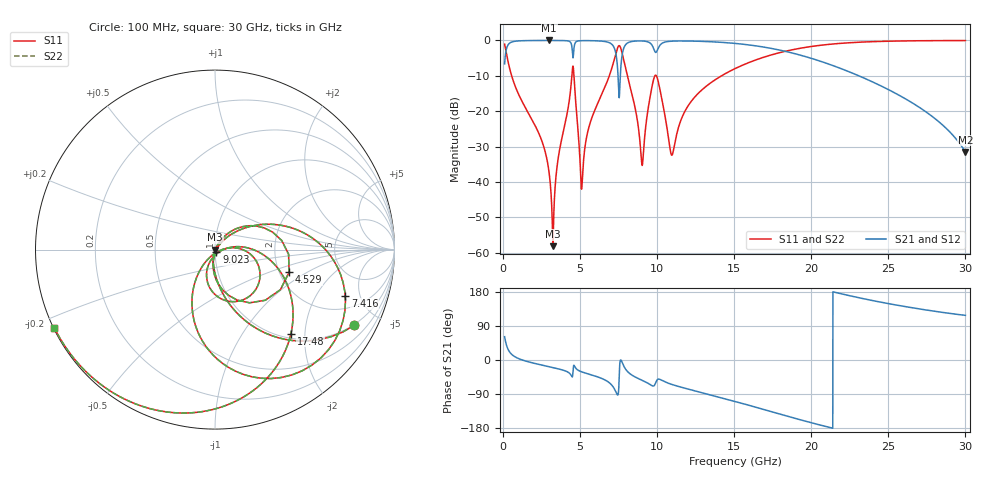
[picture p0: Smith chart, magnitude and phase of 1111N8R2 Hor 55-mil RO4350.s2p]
# GHz S MA R 50
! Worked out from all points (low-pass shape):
!   3201 points, 100 MHz to 30 GHz, reference 50 ohm
!   highest |S21| = -0.01 dB at 2.997 GHz (marker M1); lowest = -31.5 dB at 30 GHz (marker M2)
!   |S21| within 3 dB of the highest: 189.1 MHz to 4.496 GHz (4.307 GHz wide, 184 % of centre); 9.986 GHz to 18.24 GHz (8.255 GHz wide, 58.5 % of centre)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
!   lowest |S11| = -58.1 dB at 3.24 GHz (marker M3), VSWR 1.00, Z = 50.1 - j0.0199 ohm
!   |S11| at or under -10 dB: 557.3 MHz to 4.463 GHz (3.906 GHz wide, 156 % of centre); 4.6 GHz to 6.894 GHz (2.294 GHz wide, 39.9 % of centre); 9.95 GHz to 14.17 GHz (4.224 GHz wide, 35 % of centre)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
!   |S22| runs from -58.1 to 0.0 dB; largest |S21 - S12| = 0
!   S11 on the Smith chart (normalised r, x): 100 MHz: 0.96, -3.71; 4.529 GHz: 2.26, -0.70; 7.416 GHz: 2.87, -3.64; 9.023 GHz: 1.02, -0.03; 17.48 GHz: 1.09, -1.70; 30 GHz: 0.00, -0.23
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0.1  0.884 -28.5  0.4671 61.5  0.4671 61.5  0.884 -28.5
0.6793125  0.2615 -79.0  0.9647 10.9  0.9647 10.9  0.2615 -79.0
2.996563  0.01309 -103.2  0.9985 -17.8  0.9985 -17.8  0.01309 -103.2
3.2395  0.001243 -9.2  0.9984 -20.0  0.9984 -20.0  0.001243 -9.2
3.603906  0.02366 62.1  0.9975 -23.5  0.9975 -23.5  0.02366 62.1
4.528937  0.4318 -17.0  0.5808 -35.7  0.5808 -35.7  0.4318 -17.0
5.089563  0.007942 -30.4  0.9915 -31.1  0.9915 -31.1  0.007942 -30.4
5.6315  0.06628 47.8  0.9924 -38.0  0.9924 -38.0  0.06628 47.8
7.005031  0.3734 21.8  0.9004 -64.1  0.9004 -64.1  0.3734 21.8
7.416156  0.7703 -19.6  0.4435 -91.8  0.4435 -91.8  0.7703 -19.6
7.64975  0.7616 -70.3  0.4378 -0.1  0.4378 -0.1  0.7616 -70.3
7.930063  0.4189 -105.9  0.8572 -22.9  0.8572 -22.9  0.4189 -105.9
9.023281  0.01712 -60.9  0.982 -53.5  0.982 -53.5  0.01712 -60.9
9.696031  0.2407 -16.0  0.8335 -68.4  0.8335 -68.4  0.2407 -16.0
10.06978  0.2616 -87.1  0.7767 -50.4  0.7767 -50.4  0.2616 -87.1
10.96678  0.02405 -47.2  0.9758 -64.7  0.9758 -64.7  0.02405 -47.2
12.2095  0.1379 6.8  0.9787 -78.9  0.9787 -78.9  0.1379 6.8
15.05  0.3995 -20.4  0.9073 -109.3  0.9073 -109.3  0.3995 -20.4
17.47938  0.6307 -47.8  0.7655 -137.1  0.7655 -137.1  0.6307 -47.8
20.03956  0.8233 -76.6  0.5552 -166.0  0.5552 -166.0  0.8233 -76.6
25.01978  0.9746 -121.9  0.2013 148.7  0.2013 148.7  0.9746 -121.9
30  0.9956 -153.9  0.02662 117.9  0.02662 117.9  0.9956 -153.9
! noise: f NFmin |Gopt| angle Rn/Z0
0.1  0.001192  0.8462  2.179  0.001647
3.417  0.009879  0.4822  20.88  0.003162
6.743  0.04098  0.7202  39.88  0.02572
10.06  0.2196  0.9149  59.41  0.4295
13.39  0.04583  0.566  74.71  0.01257
16.7  0.0548  0.5672  87.33  0.01279
20.03  0.07885  0.6518  101.4  0.01842
23.35  0.1327  0.7718  118.1  0.03283
26.67  0.2858  0.8877  136.3  0.07824
30  1.288  0.9739  154.3  0.5667
